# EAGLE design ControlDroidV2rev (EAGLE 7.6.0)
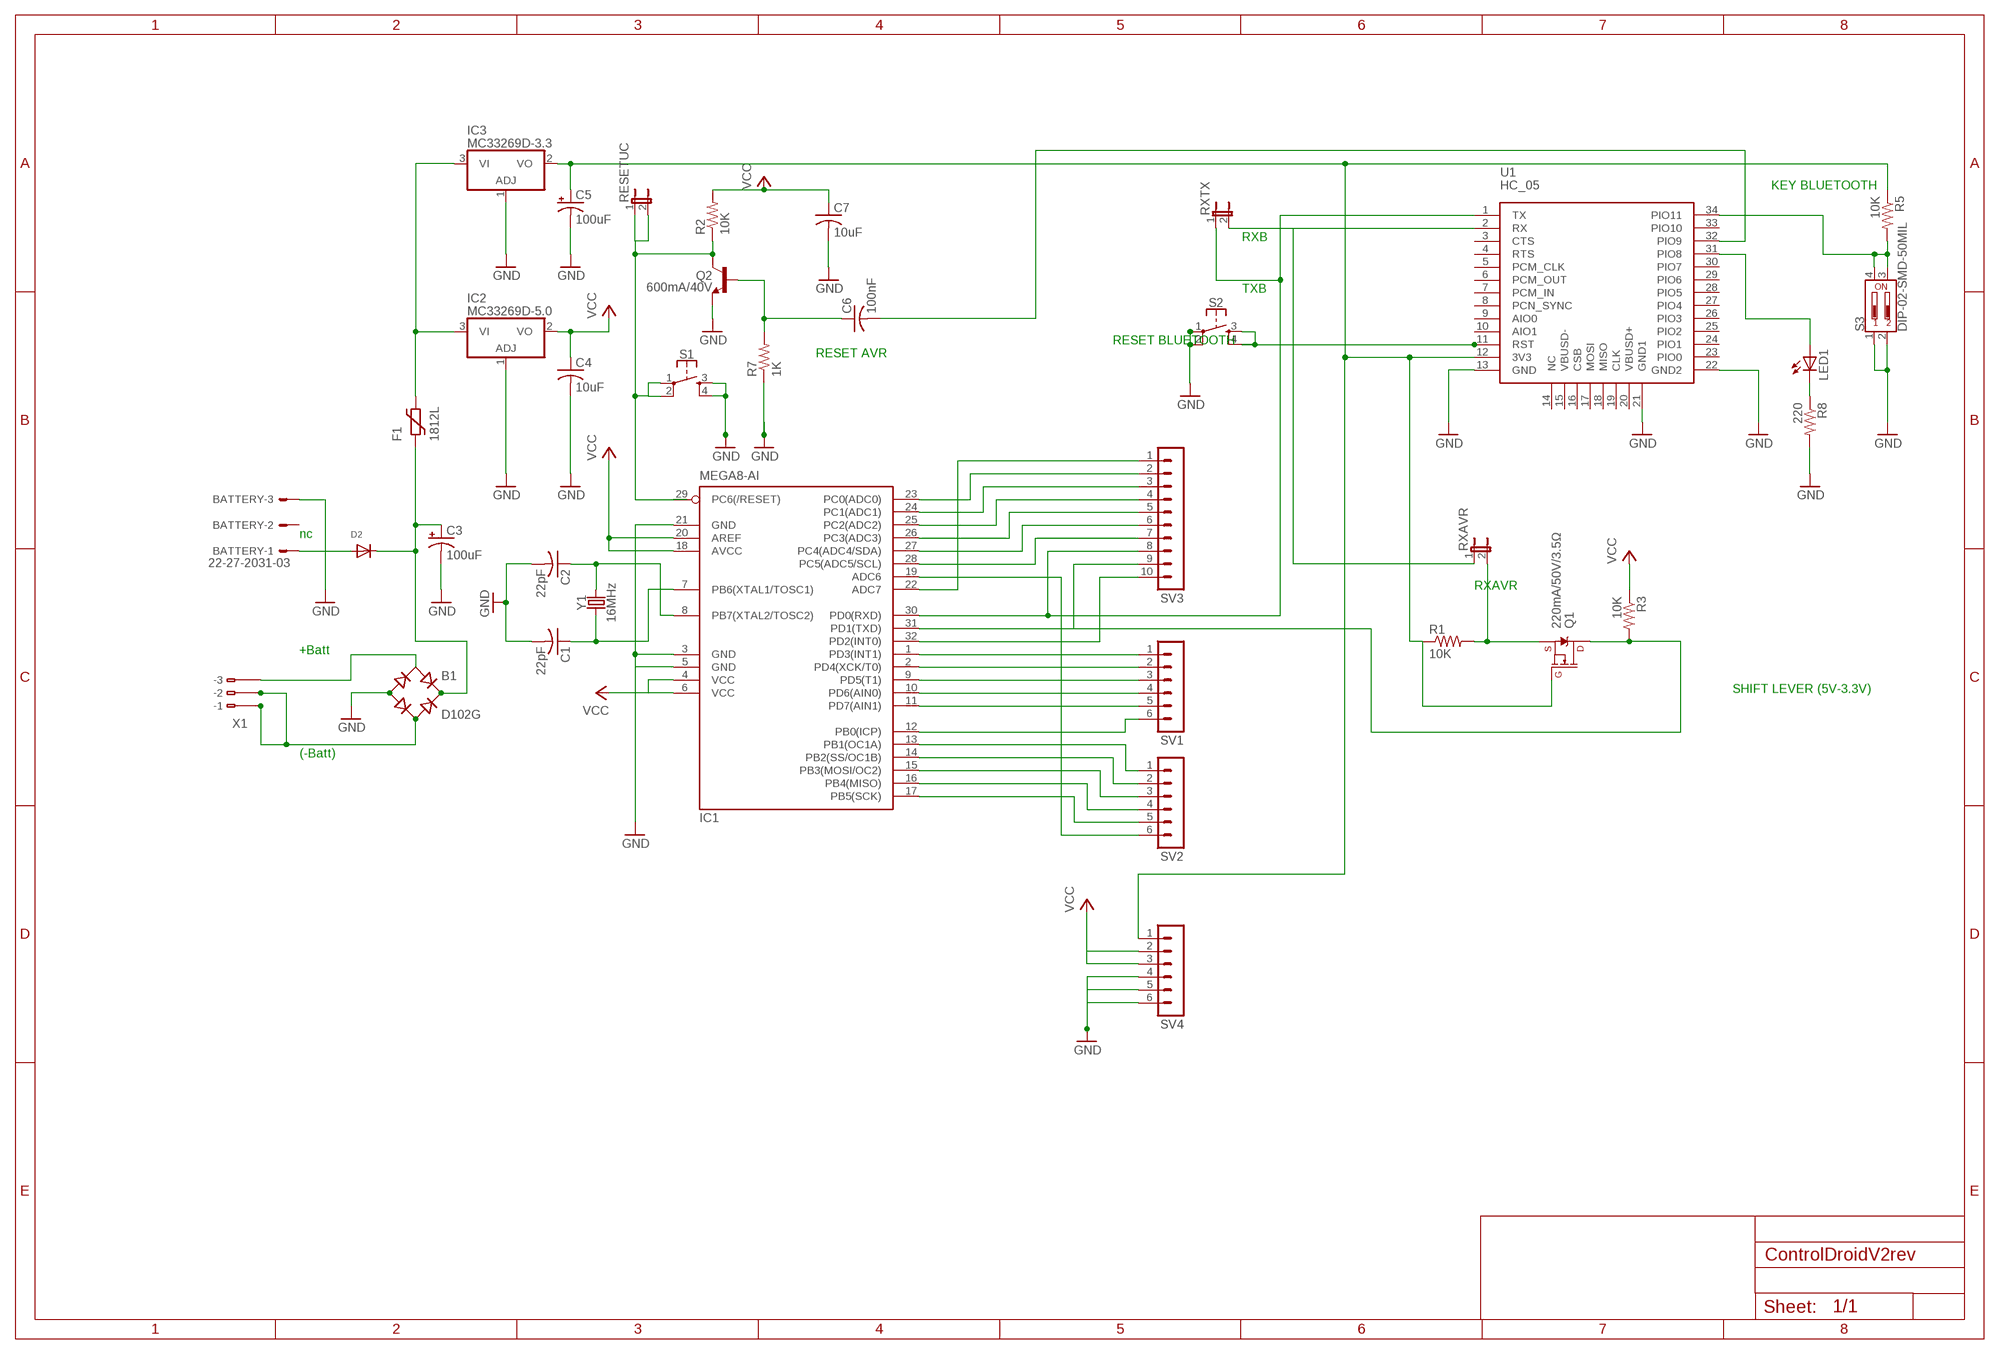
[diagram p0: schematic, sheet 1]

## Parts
B1  D102G  DBS102G  [DBS]
BATTERY  22-27-2031-03  [6410-03]
C1  22pF  C-USC1206  [C1206]
C2  22pF  C-USC1206  [C1206]
C3  100uF  CPOL-US153CLV-0605  [153CLV-0605]
C4  10uF  C-USC1206  [C1206]
C5  100uF  CPOL-US153CLV-0605  [153CLV-0605]
C6  100nF  C-USC0805  [C0805]
C7  10uF  C-USC1206  [C1206]
D2  DIODE_SOD-123FL  [SOD-123FL]
F1  1812L  [1812L]
IC1  MEGA8-AI  [TQFP32-08]
IC2  MC33269D-5.0  [DPACK]
IC3  MC33269D-3.3  [DPACK]
LED1  LEDSMT1206  [1206]
Q1  220mA/50V/3.5Ω  MOSFET-NCH-BSS138  [SOT23-3]
Q2  600mA/40V  TRANS_NPN-MMBT2222AL  [SOT23-3]
R1  10K  R-US_R1206  [R1206]
R2  10K  R-US_R1206  [R1206]
R3  10K  R-US_R1206  [R1206]
R5  10K  R-US_R1206  [R1206]
R7  1K  R-US_R1206  [R1206]
R8  220  R-US_R1206  [R1206]
RESETUC  JP1E  [JP1]
RXAVR  JP1E  [JP1]
RXTX  JP1E  [JP1]
S1  MOMENTARY-SWITCH-SPST-2-SMD-5.2MM  [TACTILE_SWITCH_SMD_5.2MM]
S2  MOMENTARY-SWITCH-SPST-2-SMD-5.2MM  [TACTILE_SWITCH_SMD_5.2MM]
S3  DIP-02-SMD-50MIL  [DIPSWITCH-02-50MIL]
SV1  MA06-1  [MA06-1]
SV2  MA06-1  [MA06-1]
SV3  MA10-1  [MA10-1]
SV4  MA06-1  [MA06-1]
U1  HC_05  [BLUETOOTH_SMD]
X1  233-103  [233-103]
Y1  16MHz  CRYSTALSMD-HC49UP  [HC49UP]

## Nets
GND: B1.- BATTERY.3 C1.2 C2.2 C3.- C4.2 C5.- C7.2 IC1.3(GND) IC1.5(GND) IC1.21(GND) IC2.1(ADJ) IC3.1(ADJ) Q2.2(E) R7.1 R8.2 S1.3 S1.4 S2.1 S2.2 S3.1 S3.2 SV4.4 SV4.5 SV4.6 U1.13(GND) U1.21(GND1) U1.22(GND2)
N$1: C1.1 IC1.7(PB6(XTAL1/TOSC1)) Y1.1
N$2: C2.1 IC1.8(PB7(XTAL2/TOSC2)) Y1.2
N$3: IC1.1(PD3(INT1)) SV1.1
N$4: IC1.2(PD4(XCK/T0)) SV1.2
N$5: IC1.9(PD5(T1)) SV1.3
N$6: IC1.10(PD6(AIN0)) SV1.4
N$7: IC1.11(PD7(AIN1)) SV1.5
N$8: IC1.12(PB0(ICP)) SV1.6
N$9: IC1.13(PB1(OC1A)) SV2.1
N$10: IC1.14(PB2(SS/OC1B)) SV2.2
N$11: IC1.15(PB3(MOSI/OC2)) SV2.3
N$12: IC1.16(PB4(MISO)) SV2.4
N$13: IC1.17(PB5(SCK)) SV2.5
N$14: IC1.19(ADC6) SV2.6
N$15: IC1.22(ADC7) SV3.1
N$16: IC1.23(PC0(ADC0)) SV3.2
N$17: IC1.24(PC1(ADC1)) SV3.3
N$18: IC1.25(PC2(ADC2)) SV3.4
N$19: IC1.26(PC3(ADC3)) SV3.5
N$20: IC1.27(PC4(ADC4/SDA)) SV3.6
N$21: IC1.28(PC5(ADC5/SCL)) SV3.7
N$22: IC1.30(PD0(RXD)) RXTX.1 SV3.8 U1.1(TX)
N$23: IC1.31(PD1(TXD)) Q1.3(D) R3.2 SV3.9
N$24: IC1.32(PD2(INT0)) SV3.10
N$30: B1.AC1 X1.B3(B-3)
N$31: C6.1 Q2.1(B) R7.2
N$32: Q1.2(S) R1.2 RXAVR.2
N$33: IC1.29(PC6(/RESET)) Q2.3(C) R2.1 RESETUC.1 RESETUC.2 S1.1 S1.2
N$34: B1.+ C3.+ D2.C F1.P$1
N$35: C5.+ IC3.2(VO) Q1.1(G) R1.1 R5.1 SV4.1 U1.12(3V3)
N$36: RXAVR.1 RXTX.2 U1.2(RX)
N$37: R5.2 S3.3 S3.4 U1.34(PIO11)
N$38: F1.P$2 IC2.3(VI) IC3.3(VI)
N$39: C6.2 U1.32(PIO9)
N$41: LED1.A U1.31(PIO8)
N$42: LED1.C R8.1
N$43: S2.3 S2.4 U1.11(RST)
N$44: BATTERY.1 D2.A
N$45: B1.AC2 X1.B1(B-1) X1.B2(B-2)
VCC: C4.1 C7.1 IC1.4(VCC) IC1.6(VCC) IC1.18(AVCC) IC1.20(AREF) IC2.2(VO) R2.2 R3.1 SV4.2 SV4.3
Unconnected: BATTERY.2 U1.3(CTS) U1.4(RTS) U1.5(PCM_CLK) U1.6(PCM_OUT) U1.7(PCM_IN) U1.8(PCN_SYNC) U1.9(AIO0) U1.10(AIO1) U1.14(NC) U1.15(VBUSD-) U1.16(CSB) U1.17(MOSI) U1.18(MISO) U1.19(CLK) U1.20(VBUSD+) U1.23(PIO0) U1.24(PIO1) U1.25(PIO2) U1.26(PIO3) U1.27(PIO4) U1.28(PIO5) U1.29(PIO6) U1.30(PIO7) U1.33(PIO10) X1.A1(-1) X1.A2(-2) X1.A3(-3)

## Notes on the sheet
- KEY BLUETOOTH
- RXB
- TXB
- RESET BLUETOOTH
- RESET AVR
- nc
- RXAVR
- +Batt
- SHIFT LEVER (5V-3.3V)
- (-Batt)

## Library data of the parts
B1 = rectifier:DB?*G: Single Phase 1.0 AMP Glass Passivated Bridge Rectifier Taiwan Semiconductor Co.,Ltd. - TSC Source: http://www.taiwansemi.com/TSCbig5/ezcatfiles/cust/img/img/db101g.pdf http://www.ts.com.tw/db/pictures/modules/PDT/PDT060207001/DBLS201G.pdf
BATTERY = con-molex:22-?-03: CONNECTOR wire to board 2.54 mm (.1 inch) pitch header; OC_FARNELL: unknown; OC_NEWARK: unknown
C1 C2 C4 C6 C7 = resistor:C-US: CAPACITOR, American symbol
C3 C5 = resistor:CPOL-US: POLARIZED CAPACITOR, American symbol
D2 = adafruit:DIODE: Diode
F1 = ptc-littlefuse:1812L
IC1 = atmel:MEGA8: MICROCONTROLLER 8 Kbytes FLASH, 1 kbytes SRAM, 512 bytes EEPROM, USART, 6-channel 10 bit ADC, 2-channel 8 bit ADC Pin compatible with Atmega48, ATMega88, ATMega168 Source: avr.lbr; MPN: ATMEGA8-16AU; OC_FARNELL: 9171371; OC_NEWARK: 73M8863
IC2 IC3 = linear:MC33269?*: Adjustable Output Low Dropout Voltage Regulator 800 mA Source: http://www.onsemi.com/pub/Collateral/MC33269-D.PDF
LED1 = adafruit:LED: LED
Q1 = SparkFun-DiscreteSemi:MOSFET-NCH: N-channel MOSFETs Voltage controlled devices that allow control of high current outputs. SparkFun Products: SparkFun OpenScale SparkFun Digital Sandbox SparkFun Monster Moto Shield SparkFun MOSFET Power Controller; PROD_ID: TRANS-00830
Q2 = SparkFun-DiscreteSemi:TRANS_NPN: NPN transistor Current controlled devices typically used to amplify current or used as a switch. BC547 - COM-08928 (TO-92 45V 100mA) (1.Collector 2.Base 3.Emitter) 2N3904 - COM-00521 (TO-92 40V 200mA) (1.Emitter 2.Base 3.Collector) P2N2222A - COM-12852 (TO-92 40V 600mA) (1.Collector 2.Base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; PROD_ID: TRANS-08049
R1-R3 R5 R7 R8 = resistor:R-US_: RESISTOR, American symbol
RESETUC RXAVR RXTX = jumper:JP1E: JUMPER
S1 S2 = SparkFun-Switches:MOMENTARY-SWITCH-SPST-2: Momentary Switch (Pushbutton) - SPST - Two Circuits Normally-open (NO) SPST momentary switches (buttons, pushbuttons). Schematic symbol includes two switch circuits. Variants SMD-4.6MMX2.8MM - 4.60mm x 2.80mm Tactile Momentary Button Switch - Used on SparkFun SAMD21 Mini Breakout SMD-5.2MM - Mini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; PROD_ID: SWCH-08247; SF_SKU: COM-08720
S3 = SparkFun-Switches:DIP-02: 2-Position DIP Switch 2-circuit DIP (dual inline package) switch. Commonly used to physcially set a circuit's behavior. Variants PTH-100MIL - Through-hole, 0.1"-Pitch Used on SparkFun Stepoko (ROB-13899) SMD-50MIL-JWING - SMD (J-Wing Pads), 0.05"-Pitch Prototype Part SMD-50MIL - SMD, 0.05"-Pitch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; PROD_ID: SWCH-13215
SV1 SV2 SV4 = con-lstb:MA06-1: PIN HEADER; OC_FARNELL: unknown; OC_NEWARK: unknown
SV3 = con-lstb:MA10-1: PIN HEADER; OC_FARNELL: unknown; OC_NEWARK: unknown
U1 = Bluetooth HC-05:HC_05: HC-05 Bluetooth Module
X1 = con-wago:233-103: WAGO Cage Clamp; MPN: 233-103; OC_FARNELL: unknown; OC_NEWARK: 28K9045
Y1 = SparkFun-Clocks:CRYSTAL: Crystals (Generic)

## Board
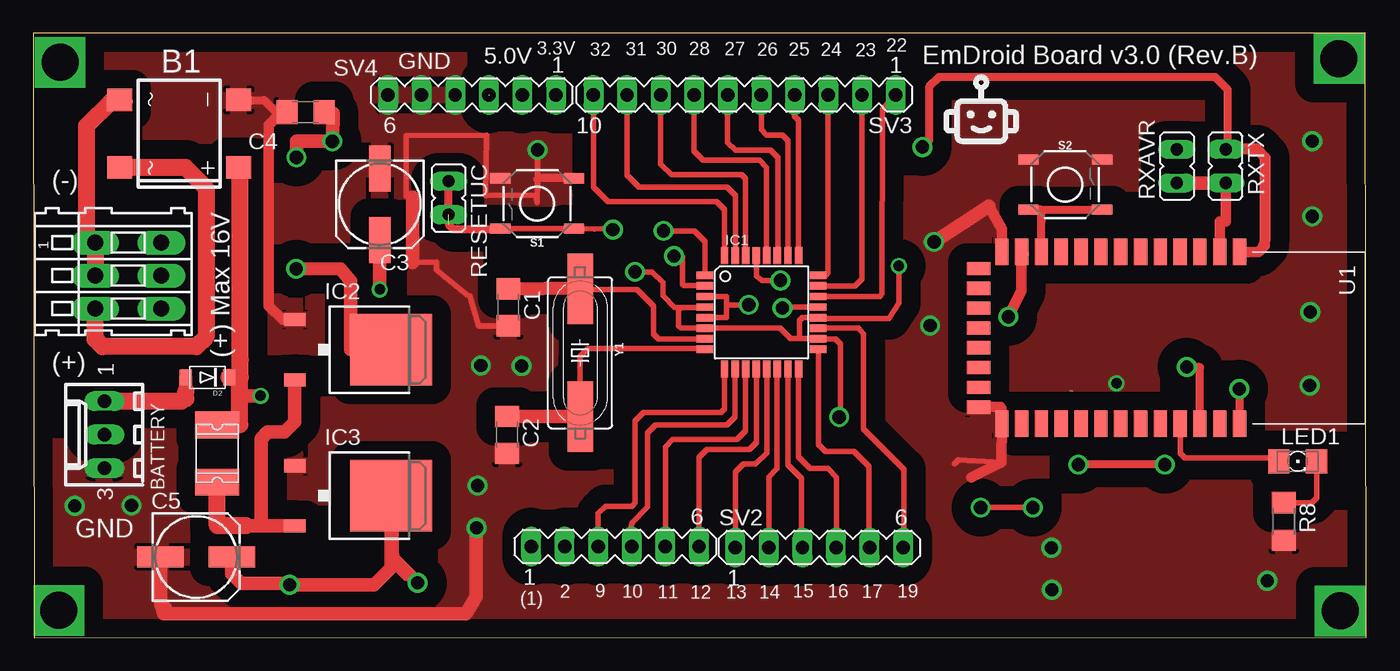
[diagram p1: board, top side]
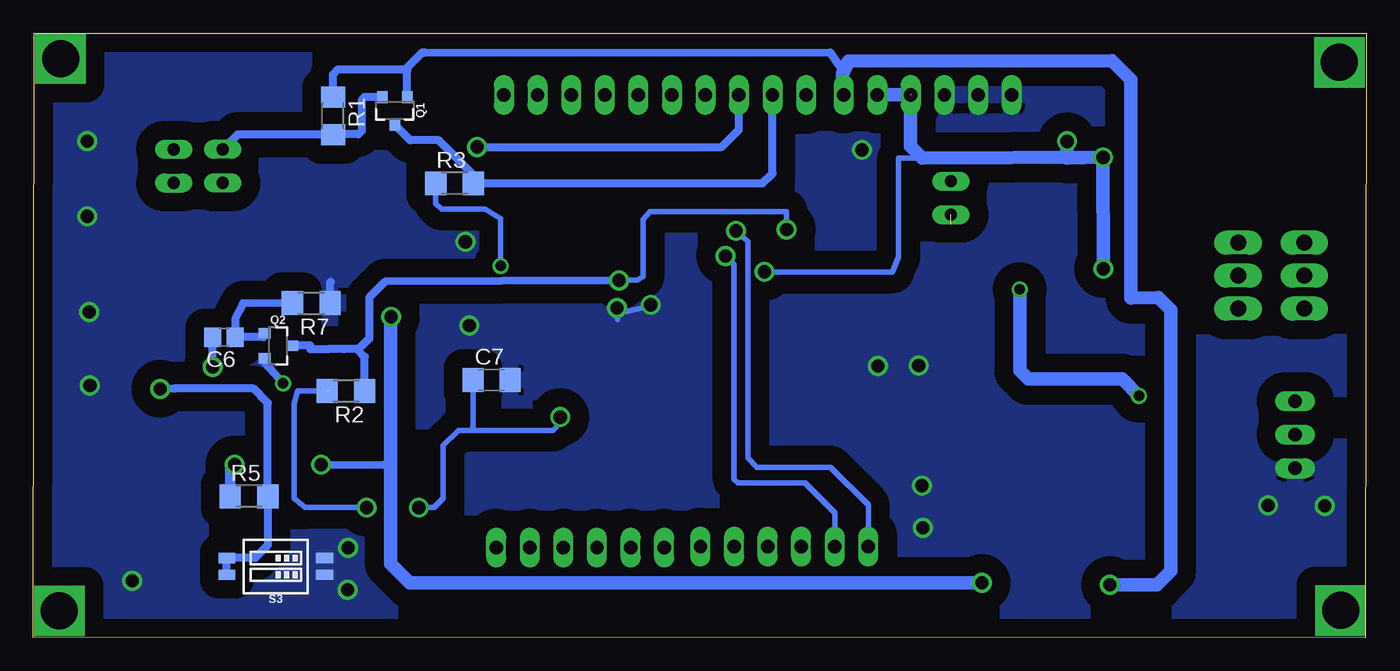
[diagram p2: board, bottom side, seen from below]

Size 100.91 x 45.78 mm. Coordinates in mm from the lower left corner, seen from the top.
Outline: 0.09,0 100.92,0.04 100.81,45.75 0,45.78 0.09,0
Copper layers (1*16): Top 0.035mm / dielectric 1.5mm / Bottom 0.035mm
Design rules "default": minimum track width 10mil, minimum drill 24mil, track to track 8mil, track to pad 8mil, pad to pad 8mil, via to via 8mil, smd to smd 8mil, copper to edge 40mil, drill to drill 8mil, minimum pad ring 10mil, minimum via ring 8mil, stop-mask expansion 4mil, vias tented up to drill 0mil, thermal gap 10mil

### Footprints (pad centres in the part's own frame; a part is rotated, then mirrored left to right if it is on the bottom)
DBS = smd 1.7 x 1.9: + -2.55,-4.5; - 2.55,-4.5; AC1 -2.55,4.5; AC2 2.55,4.5
6410-03 = drill 1.016 long: 1 2.54,0; 2 0,0; 3 -2.54,0
C1206 = smd 1.6 x 1.8: 1 -1.4,0; 2 1.4,0
153CLV-0605 = smd 3.5 x 1.6: + 2.7,0; - -2.7,0
C0805 = smd 1.3 x 1.5: 1 -0.85,0; 2 0.85,0
SOD-123FL = smd 0.91 x 1.22: A 1.637,0; C -1.637,0
1812L = smd 2.03 x 3.3: P$1 -2.16,0; P$2 2.16,0
TQFP32-08 = smd 1.27 x 0.559: 1 -4.293,2.8; 2 -4.293,2; 3 -4.293,1.2; 4 -4.293,0.4; 5 -4.293,-0.4; 6 -4.293,-1.2; 7 -4.293,-2; 8 -4.293,-2.8; 17 4.293,-2.8; 18 4.293,-2; 19 4.293,-1.2; 20 4.293,-0.4; 21 4.293,0.4; 22 4.293,1.2; 23 4.293,2; 24 4.293,2.8 | smd 0.559 x 1.27: 9 -2.8,-4.293; 10 -2,-4.293; 11 -1.2,-4.293; 12 -0.4,-4.293; 13 0.4,-4.293; 14 1.2,-4.293; 15 2,-4.293; 16 2.8,-4.293; 25 2.8,4.293; 26 2,4.293; 27 1.2,4.293; 28 0.4,4.293; 29 -0.4,4.293; 30 -1.2,4.293; 31 -2,4.293; 32 -2.8,4.293
DPACK = smd 1 x 1.6: 1 -2.28,-4.8; 3 2.28,-4.8 | smd 5.4 x 6.2: 2 0,2.5
1206 = smd 1.6 x 1.803: A -1.422,0; C 1.422,0
SOT23-3 = smd 0.8 x 0.9: 1 -0.95,-1; 2 0.95,-1; 3 0,1.1
R1206 = smd 1.6 x 1.803: 1 -1.422,0; 2 1.422,0
JP1 = drill 0.914 long: 1 0,-1.27; 2 0,1.27
TACTILE_SWITCH_SMD_5.2MM = smd 1.524 x 0.762: 1 -2.794,1.905; 2 2.794,1.905; 3 -2.794,-1.905; 4 2.794,-1.905
DIPSWITCH-02-50MIL = smd 0.762 x 1.27: 1 -0.635,-3.7; 2 0.635,-3.7; 3 0.635,3.7; 4 -0.635,3.7
MA06-1 = drill 1.016 long: 1 -6.35,0; 2 -3.81,0; 3 -1.27,0; 4 1.27,0; 5 3.81,0; 6 6.35,0
MA10-1 = drill 1.016 long: 1 -11.43,0; 2 -8.89,0; 3 -6.35,0; 4 -3.81,0; 5 -1.27,0; 6 1.27,0; 7 3.81,0; 8 6.35,0; 9 8.89,0; 10 11.43,0
BLUETOOTH_SMD = smd 2 x 1: 1 -6.35,3.81; 2 -6.35,2.31; 3 -6.35,0.81; 4 -6.35,-0.69; 5 -6.35,-2.19; 6 -6.35,-3.69; 7 -6.35,-5.19; 8 -6.35,-6.69; 9 -6.35,-8.19; 10 -6.35,-9.69; 11 -6.35,-11.19; 12 -6.35,-12.69; 13 -6.35,-14.19; 22 6.65,-14.19; 23 6.65,-12.69; 24 6.65,-11.19; 25 6.65,-9.69; 26 6.65,-8.19; 27 6.65,-6.69; 28 6.65,-5.19; 29 6.65,-3.69; 30 6.65,-2.19; 31 6.65,-0.69; 32 6.65,0.81; 33 6.65,2.31; 34 6.65,3.81 | smd 1 x 1.8: 14 -5.1,-15.94; 15 -3.6,-15.94; 16 -2.1,-15.94; 17 -0.6,-15.94; 18 0.9,-15.94; 19 2.4,-15.94; 20 3.9,-15.94; 21 5.4,-15.94
233-103 = drill 1.2 long: A1 -2.5,2.5; A2 0,2.5; A3 2.5,2.5; B1 -2.5,-2.5; B2 0,-2.5; B3 2.5,-2.5
HC49UP = smd 5.334 x 1.93: 1 -4.826,0; 2 4.826,0

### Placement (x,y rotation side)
B1  11.05,38.16 90 top
BATTERY  5.39,15.37 90 top
C1  35.97,25.01 270 top
C2  35.87,15.36 270 top
C3  26.24,32.81 270 top
C4  20.63,39.78 180 top
C5  12.34,6.11 0 top
C6  86.46,22.75 180 bottom
C7  66.21,19.5 0 bottom
D2  13.2,19.71 180 top
F1  13.94,13.94 270 top
IC1  55.13,24.63 0 top
IC2  24.61,21.8 270 top
IC3  24.61,10.75 270 top
LED1  95.71,13.35 0 top
Q1  73.54,39.93 180 bottom
Q2  82.38,22.1 270 bottom
R1  78.21,39.51 270 bottom
R2  77.23,18.69 180 bottom
R3  69.01,34.4 0 bottom
R5  84.56,10.7 0 bottom
R7  79.86,25.33 180 bottom
R8  94.66,8.8 270 top
RESETUC  31.45,33.29 180 top
RXAVR  86.56,35.7 0 top
RXTX  90.26,35.7 180 top
S1  38.15,32.87 180 top
S2  78.11,34.3 0 top
S3  82.54,5.39 90 bottom
SV1  44.05,6.9 0 top
SV2  59.5,6.83 0 top
SV3  53.84,41.09 180 top
SV4  33.21,41.1 180 top
U1  87.5,22.85 270 top
X1  7.21,27.41 270 top
Y1  41.4,21.57 270 top

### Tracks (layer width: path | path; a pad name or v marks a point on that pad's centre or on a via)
GND  (via drill 0.8, 1)
  Top 0.406: IC1.3 52.48,25.83 52.46,25.2 | 52.46,25.2 52.46,24.25 50.86,24.25 IC1.5 | 52.46,25.2 v54.16,25.2 | IC1.21 56.98,25.03 v56.71,24.95 | v38.17,36.93 38.17,34.68 38.16,32.95 38.06,33.5 34.23,33.47 34.33,38.06 28.22,38.01 28.22,33.42 28.71,33.37 28.26,33.49 | 28.71,28.39 30.55,28.44 30.55,27.83 32.81,25.97 33.02,25.85 33.06,25.84 33.71,23.6 C1.2 | 73.27,13.28 70.02,13.46 69.71,13.15
  Top 0.61: v81.99,19.25 82.1,19.56 82.01,19.47 | S1.3 38.26,34.78 38.17,34.68 | C4.2 18.77,39.75 18.6,39.58 17.47,40.71 B1.-
  Top 0.813: U1.13 73.31,30.93 72.32,32.66 | 71.01,12.15 73.27,13.28 U1.22 73.3,17.34 73.19,17.45 U1.21 | IC2.1 18.87,24.08 17.83,25.12 17.83,38.81 18.6,39.58
  Top 1.016: 28.71,33.37 28.71,28.39 | 72.32,32.66 v68.19,29.97 | 10,2.26 9.64,2.62 C5.- 9.64,2.54 9.88,1.8 32.76,1.8 33.55,3.1 33.55,8.3 v33.56,8.31
  Bottom 0.406: v54.16,25.2 54.71,25 55.96,24.7 v56.71,24.95 56.91,25.05 56.66,24.1
  Bottom 0.61: R7.1 78.44,26.88 78.36,26.95 | Q2.2 83.38,20.81 v81.99,19.25
  other vias: 3.16,9.99 33.64,11.51 33.88,20.6 36.96,20.57 96.66,24.65 93.41,4.3 96.81,31.9 77.08,6.8 77.11,3.63 96.61,19.1 7.45,10.02 96.81,37.59 67.9,23.63
  pour Top (isolate 1.422): -0.65,45.44 100.31,46.49 99.74,0.64 -1.17,0.59
  pour Bottom (isolate 1.422): 1.19,45.86 100.06,46.14 100.64,0.46 1.07,0.38
N$1
  Top 0.406: IC1.7 47.33,22.63 46.96,23 46.96,25.1 45.71,26.35 41.45,26.35 Y1.1
  Top 1.016: C1.1 41.34,26.46 Y1.1
N$2
  Top 0.406: Y1.2 41.4,21.29 42.01,21.9 50.77,21.9 IC1.8
  Top 1.016: C2.1 41.39,16.76 Y1.2
N$3  (via drill 1)
  Top 0.406: v47.71,30.8 50.06,30.8 50.86,30 50.86,27.46 IC1.1
  Bottom 0.406: SV1.1 37.7,10.04 40.56,12.9 46.11,12.9 46.81,13.6 46.81,30 v47.71,30.8
N$4  (via drill 1)
  Top 0.406: v48.51,28.9 49.16,28.85 49.16,26.75 49.26,26.65 50.82,26.65 IC1.2
  Bottom 0.406: SV1.2 40.24,9.43 42.51,11.7 47.56,11.7 47.86,12 47.86,28.25 v48.51,28.9
N$5
  Top 0.406: IC1.9 52.33,17.32 52.06,17.05 46.21,17.05 45.56,16.4 45.56,10.2 45.31,9.95 43.31,9.95 42.76,9.4 42.76,6.92 SV1.3
N$6
  Top 0.406: SV1.4 45.32,8.16 45.26,8.36 45.31,8.7 46.51,9.9 46.51,15.5 47.11,16.1 52.51,16.1 53.11,16.7 53.11,20.32 IC1.10
N$7
  Top 0.406: SV1.5 47.86,14.45 48.41,15 53.26,15 53.91,15.65 53.91,20.32 IC1.11
N$8
  Top 0.406: IC1.12 54.73,14.77 54.21,14.25 51.01,14.25 50.41,13.65 SV1.6
N$9
  Top 0.406: SV2.1 53.15,12.54 53.76,13.15 54.66,13.15 55.54,14 55.54,20.32 IC1.13
N$10
  Top 0.406: SV2.2 55.69,12.18 56.31,12.8 56.31,20.32 IC1.14
N$11
  Top 0.406: IC1.15 57.13,13.08 58.16,12.05 58.16,6.9 SV2.3
N$12
  Top 0.406: IC1.16 57.93,13.68 58.81,12.8 60.16,12.8 60.81,12.15 60.81,6.87 SV2.4
N$13
  Top 0.406: IC1.17 59.43,14.64 59.96,14.1 62.11,14.1 63.26,12.95 63.26,6.88 SV2.5
N$14
  Top 0.406: IC1.19 62.48,23.43 62.86,23 62.86,15.8 65.91,12.75 65.91,6.89 SV2.6
N$15
  Top 0.406: IC1.22 64.08,25.83 64.26,26.05 64.27,40.01 65.31,41.05 SV3.1
N$16
  Top 0.406: IC1.23 62.19,26.63 62.71,27.15 62.71,41.07 SV3.2
N$17
  Top 0.406: IC1.24 59.99,27.43 60.16,27.6 60.16,41.06 SV3.3
N$18
  Top 0.406: IC1.25 57.93,39.18 57.61,39.5 57.61,41.05 SV3.4
N$19
  Top 0.406: IC1.26 57.13,37.63 56.71,38.05 55.51,38.05 55.11,38.45 SV3.5
N$20
  Top 0.406: SV3.6 52.57,37.49 53.16,36.9 55.81,36.9 56.36,36.35 56.36,28.96 IC1.27
N$21
  Top 0.406: SV3.7 50.03,36.83 50.71,36.15 54.96,36.15 55.51,35.6 55.51,28.95 IC1.28
N$22  (via drill 1)
  Top 0.406: SV3.8 47.49,35.87 48.31,35.05 53.61,35.05 53.91,34.75 53.91,28.95 IC1.30
  Top 0.61: U1.1 92.86,29.2 93.01,29.35 93.01,29.75 93.36,30.1 93.36,36.35 92.61,37.1 90.56,37.1 90.41,36.95 90.41,41.5 89.46,42.45 68.56,42.45 67.81,41.7 67.81,37.65 v67.31,37.15
  Top 0.813: RXTX.1 92.64,36.97 93.21,36.4 93.21,29.7 92.71,29.2 U1.1
  Bottom 0.61: v67.31,37.15 48.79,37.15 47.49,38.45 SV3.8
N$23
  Top 0.406: SV3.9 44.95,35.01 45.86,34.1 52.51,34.1 53.16,33.45 53.16,28.96 IC1.31
  Bottom 0.61: SV3.9 44.95,35.15 45.7,34.4 R3.2 67.59,35.04 70.2,37.65 72.36,37.65 Q1.3
N$24
  Top 0.406: SV3.10 42.41,34.1 43.51,33 51.71,33 52.31,32.4 52.31,28.95 IC1.32
N$25  (via drill 2.8)
  other vias: 2.05,43.56
N$26  (via drill 2.8)
  other vias: 1.96,2.07
N$27  (via drill 2.8)
  other vias: 98.93,2.03
N$28  (via drill 2.8)
  other vias: 98.83,43.84
N$30
  Top 1.27: B1.AC1 11.52,35.61 13.1,34.03 13.1,22.78 12.36,22.05 5.25,22.05 4.69,22.6 4.69,24.89 X1.B3
N$31
  Bottom 0.61: R7.2 85.01,25.31 85.61,24.15 C6.1 85.59,22.77 83.46,22.76 83.46,23.05 Q2.1
N$32
  Bottom 0.61: R1.2 78.72,38.09 | 78.72,38.09 85.45,38.09 RXAVR.2 | Q1.2 75.82,40.93 76.03,40.72 76.03,38.38 76.3,38.11 78.7,38.11 78.72,38.09
N$33  (via drill 1)  (1 unrouted)
  Top 0.406: IC1.29 54.73,27.38 55.16,27.05 v56.56,27.05 | S1.1 S1.2 42.51,30.95 43.17,30.97 43.86,30.97 v43.88,30.9
  Top 0.61: RESETUC.2 RESETUC.1 | 31.45,31.28 31.81,30.92 35.31,30.92 S1.2
  Bottom 0.406: v43.88,30.9 43.89,31.64 43.9,32.26 54.21,32.25 54.76,31.65 54.76,27.34 55.16,27.08 56.64,27.08 v56.56,27.05
  Bottom 0.61: v56.56,27.05 74.26,26.95 75.46,25.75 75.46,22.65 76.26,21.85 76.41,21.85 | 76.41,21.85 77.39,21.85 78.57,21.85 78.57,21.83 79.87,21.83 79.94,21.84 79.92,22.09 79.95,22.09 79.95,22.13 81.25,22.13 Q2.3 | 76.41,21.85 75.81,21.26 R2.1
N$34  (via drill 0.8)
  Top 1.016: F1.P$1 15.64,16.13 15.62,18.31 v17.22,18.31 | D2.C 15.68,19.72 | 15.67,35.02 B1.+ | C3.+ v26.24,26.37 v26.23,26.36
  Top 1.27: 15.64,16.13 15.64,19.67 D2.C | 15.68,19.72 15.69,21.05 15.67,35.02
  Bottom 1.016: v26.23,26.36 26.23,20.22 25.6,19.58 18.49,19.58 v17.22,18.31
N$35  (via drill 1)
  Top 0.61: v85.66,13.1 v79.11,13.1
  Top 0.813: v73.81,24.3 74.78,26.25 74.78,29.06 74.86,29.06 | 74.83,29.06 74.83,28.74
  Top 1.016: 27.2,5.95 27.16,6.9 | 27.16,6.9 27.16,10.7 IC3.2 27.11,5.3 25.81,4 v19.41,4 19.29,4.12 15.74,4.12 15.04,4.82 C5.+ | 27.16,6.1 27.16,5.95 28.31,4.8 | 27.16,6.9 27.16,6.1 | 27.16,6.1 v29.11,4.15 | 74.86,29.06 74.83,29.06 | 74.83,28.74 U1.12
  Bottom 0.61: 39.6,42.84 40.6,44.32 71.24,44.3 71.46,44.29 72.59,43.15 72.59,42.94 | 85.99,12.78 v85.66,13.1 | v79.11,13.1 74.31,13.08 73.86,12.7 | Q1.1 72.59,42.94 | R1.1 78.21,42.64 77.83,43.02 72.67,43.02 72.59,42.94
  Bottom 0.813: 85.99,12.78 R5.1
  Bottom 1.016: v29.11,4.15 72.41,4.15 73.86,5.6 73.86,12.7 73.86,24.15 v73.81,24.3 | v19.41,4 15.86,4 14.81,5.05 14.81,24.8 15.76,25.75 17.81,25.71 17.84,26.61 17.84,42.26 19.26,43.69 39.21,43.65 39.6,42.84 39.66,42.7 39.66,41.2 SV4.1
N$36
  Top 0.813: U1.2 89.81,31.51 90.28,31.51 90.25,31.62 90.26,32.95 RXTX.2
  Top 1.016: RXAVR.1 RXTX.2
N$37  (via drill 1)
  Top 0.61: v91.29,18.84 91.29,16.21 U1.34
  Bottom 0.61: v91.29,18.84 90.26,18.85 84.21,18.85 83.14,17.78 R5.2 83.14,7 84.09,6.04 86.23,6.04 S3.3 S3.4
N$38
  Top 1.016: IC3.3 17.01,8.47 | 17.01,8.47 16.11,8.47 | 13.94,11.86 F1.P$2 | IC2.3 19.81,16.34 19.04,15.57 17.77,15.57 17.27,15.06 17.27,8.73 17.01,8.47
  Top 1.27: 16.11,8.47 13.94,8.48 F1.P$2
N$39  (via drill 1)
  Top 0.61: U1.32 88.31,20.49 v87.32,20.49 v87.31,20.5
  Bottom 0.61: v87.31,20.5 C6.2
N$41
  Top 0.406: U1.31 86.83,13.94 87.16,13.6 94.24,13.6 LED1.A
N$42
  Top 0.406: R8.1 96.79,10.23 97.16,10.6 97.16,13.62 LED1.C
N$43
  Top 0.406: S2.3
  Top 0.61: U1.11 76.31,31.57 76.31,32.39 S2.3 | S2.3 S2.4
N$44
  Top 1.016: 11.56,18.68 D2.A
  Top 1.27: BATTERY.1 11.23,17.92 11.57,18.11 11.56,18.68
N$45
  Top 1.016: B1.AC2 7.04,40.59 5.9,40.6 | 4.02,30.25 4.66,29.86 | 4.66,29.91 4.92,29.86 X1.B1
  Top 1.27: 5.9,40.6 4.03,38.73 4.02,30.25 | 4.66,29.86 4.66,29.91 | X1.B1 X1.B2
VCC  (via drill 0.8, 1)  (2 unrouted)
  Top 0.406: 49.06,25 48.86,24.8 48.86,23.6 49.03,23.43 IC1.6 56.53,23.43 57.31,22.65 57.96,22.65 | 49.06,25 50.81,25 IC1.4 | 49.06,25 48.56,25 47.66,25.9 47.66,26.9 46.86,27.7 v45.56,27.7 | 57.96,22.65 59.41,22.65 IC1.18 60.73,22.63 61.11,22.25 61.11,16.8 v61.01,16.7 | 57.96,22.65 58.01,22.7 58.01,24 58.24,24.23 IC1.20 59.49,24.17 64.79,24.17 65.53,25.33 v65.52,28.15 | v71.71,9.85 v75.66,9.85 75.66,9.8
  Top 1.016: IC2.2 24.05,21.81 24.05,27.01 23.29,27.93 v19.92,27.93 | C4.1 22.48,39.73 22.7,39.7 22.68,37.72 v22.66,37.58 19.93,37.58 19.93,37.36 v19.93,36.37
  Bottom 0.406: v45.56,27.7 35.86,27.7 35.41,28.8 35.41,36.3 33.61,36.3 | v61.01,16.7 61.01,16.25 61.56,15.7 67.81,15.7 | 67.81,15.7 68.71,15.7 69.86,14.55 69.86,10.55 70.56,9.85 v71.71,9.85 | v75.66,9.85 80.31,9.85 81.16,10.55 81.16,17.75 80.88,18.69 79.13,18.69 78.46,18.7 78.5,18.94 | C7.1 67.61,15.9 67.81,15.7 | R3.1 70.44,32.88 70.01,32.45 66.69,32.45 65.51,31.71 65.51,28.34 v65.52,28.15
  Bottom 1.016: v19.92,27.93 v19.93,36.37 | v19.93,36.37 22.68,36.32 22.68,37.58 v22.66,37.58 | v19.93,36.37 33.61,36.3 34.51,37.2 34.51,41.07 34.49,41.07 | SV4.3 SV4.2

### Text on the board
tNames: 3.3V | 32 | 31 | 30 | 28 | 27 | 26 | 25 | 24 | 22 | EmDroid Board v3.0 (Rev.B) | GND | 5.0V | 23 | (-) | (+) Max 16V | (+) | GND | 9 | 15 | 16 | 19 | (1) | 2 | 10 | 11 | 12 | 13 | 14 | 17

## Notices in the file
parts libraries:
SparkFun-Clocks: Licensing: Creative Commons ShareAlike 4.0 International - https://creativecommons.org/licenses/by-sa/4.0
